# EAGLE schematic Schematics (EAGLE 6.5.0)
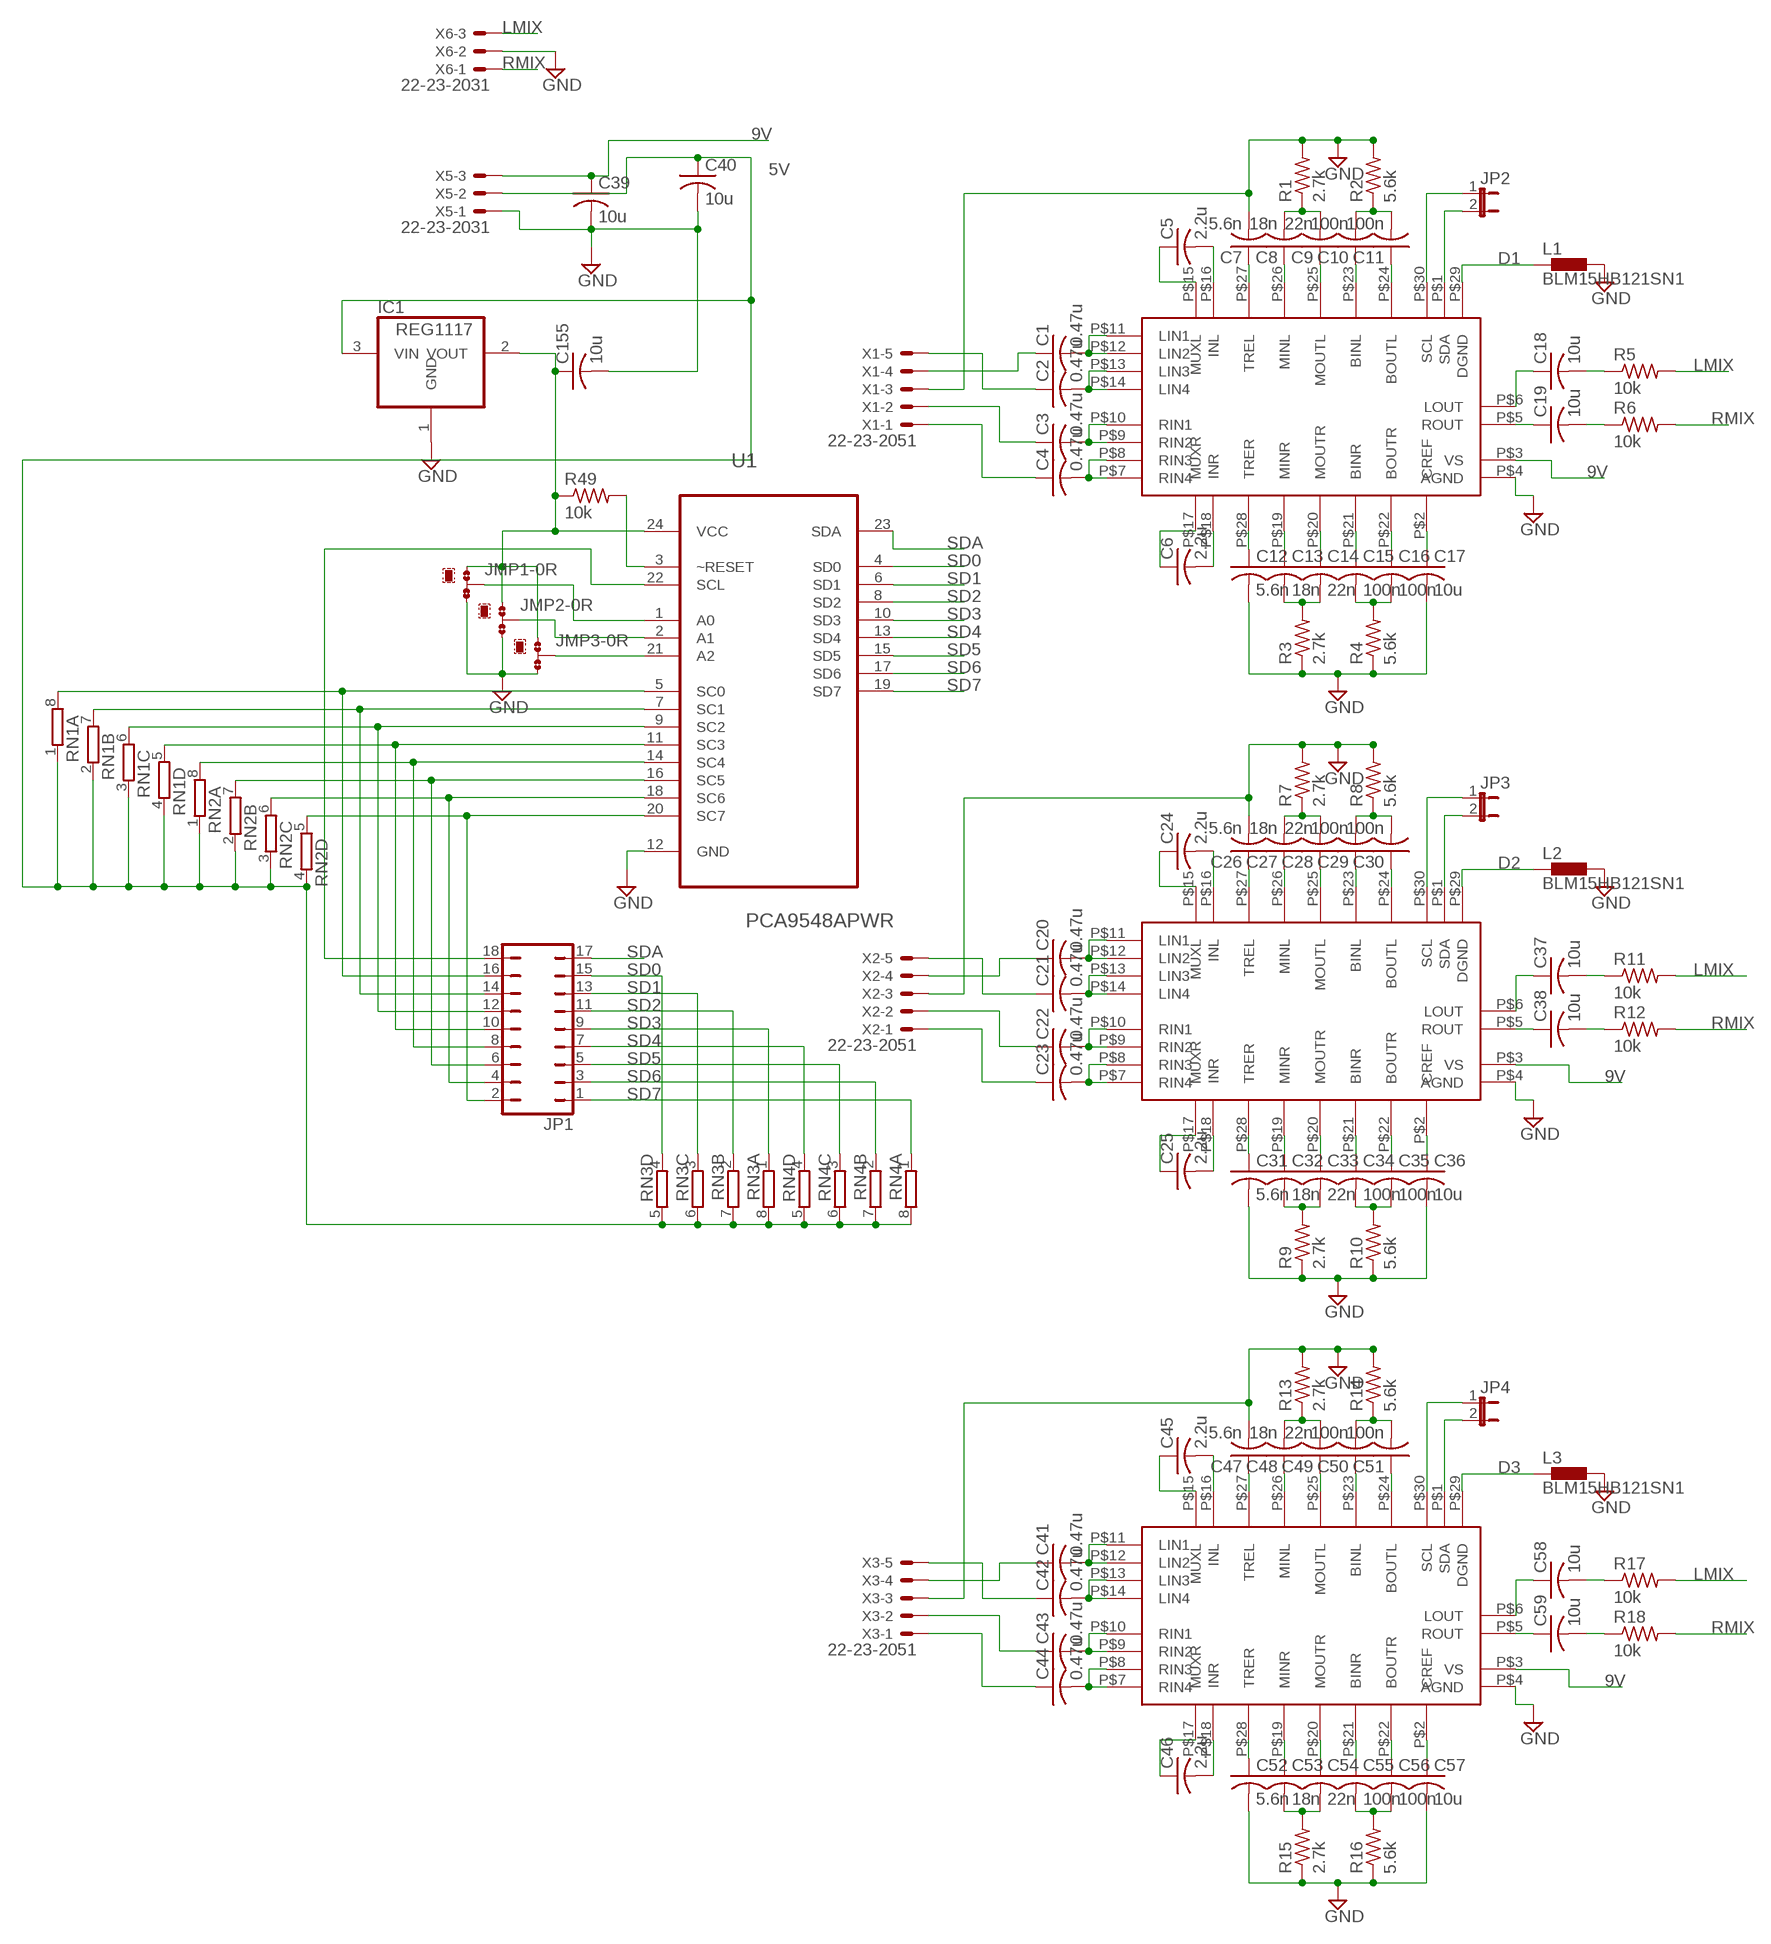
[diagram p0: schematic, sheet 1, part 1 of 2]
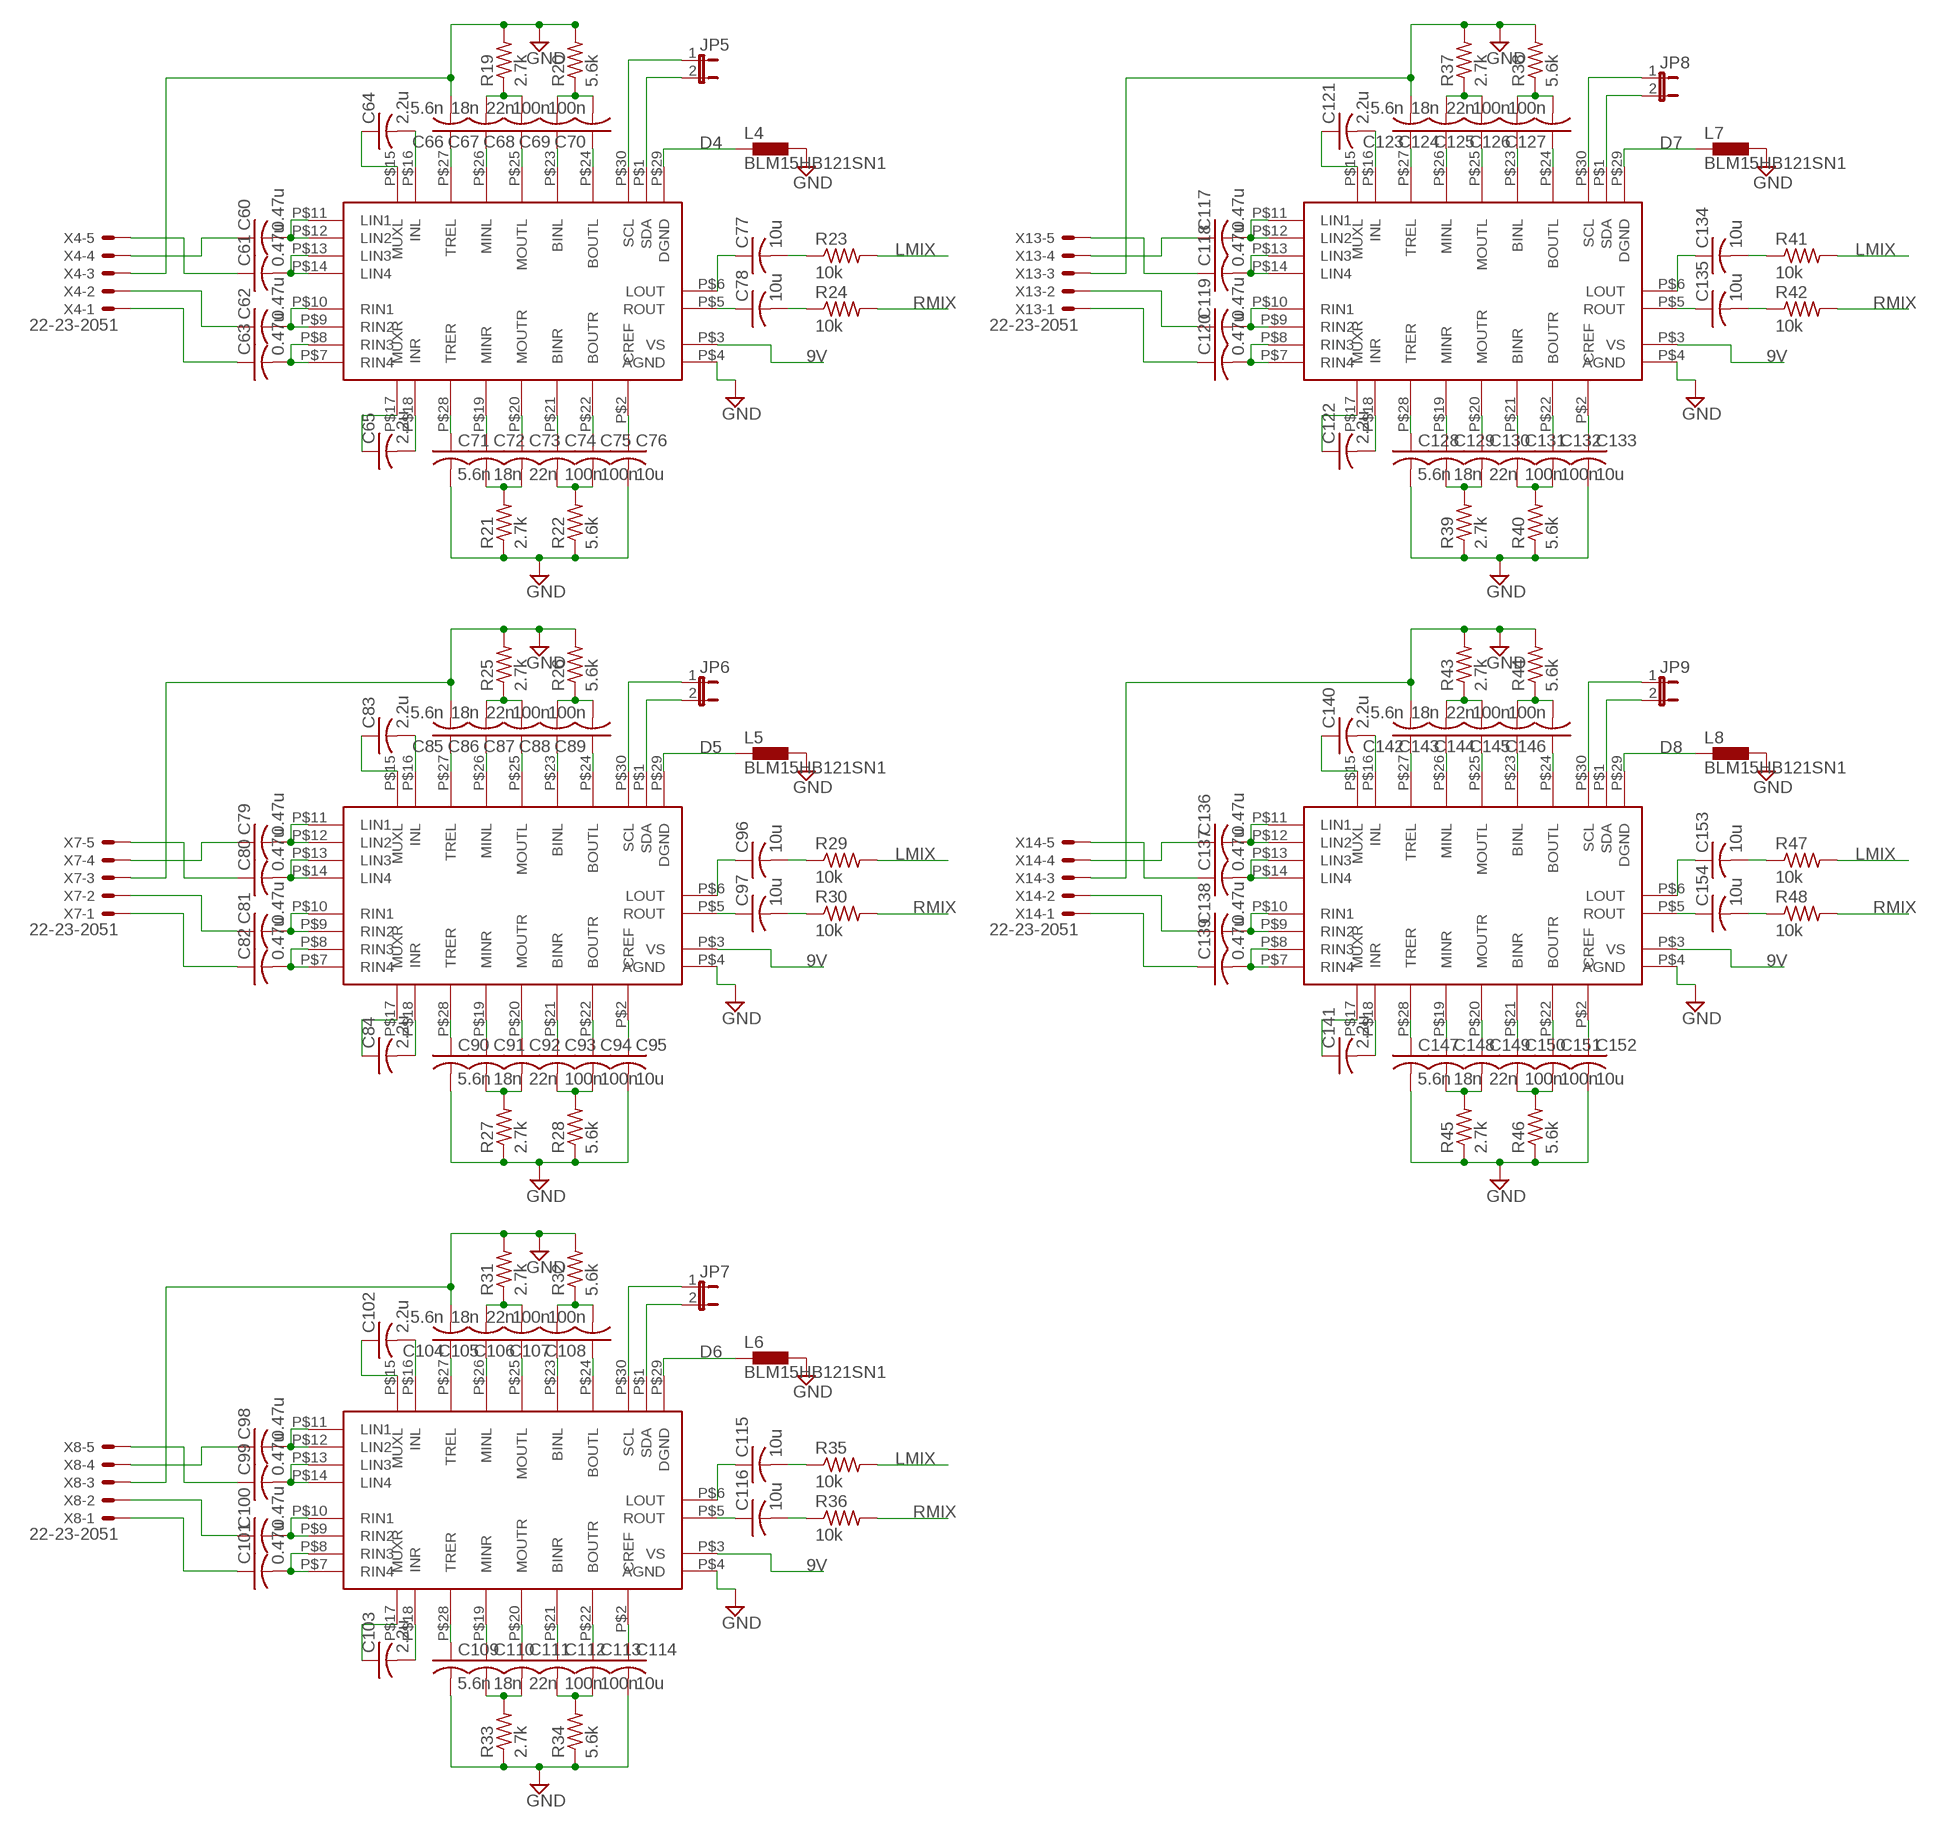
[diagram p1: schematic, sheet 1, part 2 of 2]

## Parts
C1  0.47u  C-USC1206  [C1206]
C2  0.47u  C-USC1206  [C1206]
C3  0.47u  C-USC1206  [C1206]
C4  0.47u  C-USC1206  [C1206]
C5  2.2u  C-USC1206  [C1206]
C6  2.2u  C-USC1206  [C1206]
C7  5.6n  C-USC1206  [C1206]
C8  18n  C-USC1206  [C1206]
C9  22n  C-USC1206  [C1206]
C10  100n  C-USC1206  [C1206]
C11  100n  C-USC1206  [C1206]
C12  5.6n  C-USC1206  [C1206]
C13  18n  C-USC1206  [C1206]
C14  22n  C-USC1206  [C1206]
C15  100n  C-USC1206  [C1206]
C16  100n  C-USC1206  [C1206]
C17  10u  C-USC1206  [C1206]
C18  10u  C-USC1206  [C1206]
C19  10u  C-USC1206  [C1206]
C20  0.47u  C-USC1206  [C1206]
C21  0.47u  C-USC1206  [C1206]
C22  0.47u  C-USC1206  [C1206]
C23  0.47u  C-USC1206  [C1206]
C24  2.2u  C-USC1206  [C1206]
C25  2.2u  C-USC1206  [C1206]
C26  5.6n  C-USC1206  [C1206]
C27  18n  C-USC1206  [C1206]
C28  22n  C-USC1206  [C1206]
C29  100n  C-USC1206  [C1206]
C30  100n  C-USC1206  [C1206]
C31  5.6n  C-USC1206  [C1206]
C32  18n  C-USC1206  [C1206]
C33  22n  C-USC1206  [C1206]
C34  100n  C-USC1206  [C1206]
C35  100n  C-USC1206  [C1206]
C36  10u  C-USC1206  [C1206]
C37  10u  C-USC1206  [C1206]
C38  10u  C-USC1206  [C1206]
C39  10u  C-USC1206  [C1206]
C40  10u  C-USC1206  [C1206]
C41  0.47u  C-USC1206  [C1206]
C42  0.47u  C-USC1206  [C1206]
C43  0.47u  C-USC1206  [C1206]
C44  0.47u  C-USC1206  [C1206]
C45  2.2u  C-USC1206  [C1206]
C46  2.2u  C-USC1206  [C1206]
C47  5.6n  C-USC1206  [C1206]
C48  18n  C-USC1206  [C1206]
C49  22n  C-USC1206  [C1206]
C50  100n  C-USC1206  [C1206]
C51  100n  C-USC1206  [C1206]
C52  5.6n  C-USC1206  [C1206]
C53  18n  C-USC1206  [C1206]
C54  22n  C-USC1206  [C1206]
C55  100n  C-USC1206  [C1206]
C56  100n  C-USC1206  [C1206]
C57  10u  C-USC1206  [C1206]
C58  10u  C-USC1206  [C1206]
C59  10u  C-USC1206  [C1206]
C60  0.47u  C-USC1206  [C1206]
C61  0.47u  C-USC1206  [C1206]
C62  0.47u  C-USC1206  [C1206]
C63  0.47u  C-USC1206  [C1206]
C64  2.2u  C-USC1206  [C1206]
C65  2.2u  C-USC1206  [C1206]
C66  5.6n  C-USC1206  [C1206]
C67  18n  C-USC1206  [C1206]
C68  22n  C-USC1206  [C1206]
C69  100n  C-USC1206  [C1206]
C70  100n  C-USC1206  [C1206]
C71  5.6n  C-USC1206  [C1206]
C72  18n  C-USC1206  [C1206]
C73  22n  C-USC1206  [C1206]
C74  100n  C-USC1206  [C1206]
C75  100n  C-USC1206  [C1206]
C76  10u  C-USC1206  [C1206]
C77  10u  C-USC1206  [C1206]
C78  10u  C-USC1206  [C1206]
C79  0.47u  C-USC1206  [C1206]
C80  0.47u  C-USC1206  [C1206]
C81  0.47u  C-USC1206  [C1206]
C82  0.47u  C-USC1206  [C1206]
C83  2.2u  C-USC1206  [C1206]
C84  2.2u  C-USC1206  [C1206]
C85  5.6n  C-USC1206  [C1206]
C86  18n  C-USC1206  [C1206]
C87  22n  C-USC1206  [C1206]
C88  100n  C-USC1206  [C1206]
C89  100n  C-USC1206  [C1206]
C90  5.6n  C-USC1206  [C1206]
C91  18n  C-USC1206  [C1206]
C92  22n  C-USC1206  [C1206]
C93  100n  C-USC1206  [C1206]
C94  100n  C-USC1206  [C1206]
C95  10u  C-USC1206  [C1206]
C96  10u  C-USC1206  [C1206]
C97  10u  C-USC1206  [C1206]
C98  0.47u  C-USC1206  [C1206]
C99  0.47u  C-USC1206  [C1206]
C100  0.47u  C-USC1206  [C1206]
C101  0.47u  C-USC1206  [C1206]
C102  2.2u  C-USC1206  [C1206]
C103  2.2u  C-USC1206  [C1206]
C104  5.6n  C-USC1206  [C1206]
C105  18n  C-USC1206  [C1206]
C106  22n  C-USC1206  [C1206]
C107  100n  C-USC1206  [C1206]
C108  100n  C-USC1206  [C1206]
C109  5.6n  C-USC1206  [C1206]
C110  18n  C-USC1206  [C1206]
C111  22n  C-USC1206  [C1206]
C112  100n  C-USC1206  [C1206]
C113  100n  C-USC1206  [C1206]
C114  10u  C-USC1206  [C1206]
C115  10u  C-USC1206  [C1206]
C116  10u  C-USC1206  [C1206]
C117  0.47u  C-USC1206  [C1206]
C118  0.47u  C-USC1206  [C1206]
C119  0.47u  C-USC1206  [C1206]
C120  0.47u  C-USC1206  [C1206]
C121  2.2u  C-USC1206  [C1206]
C122  2.2u  C-USC1206  [C1206]
C123  5.6n  C-USC1206  [C1206]
C124  18n  C-USC1206  [C1206]
C125  22n  C-USC1206  [C1206]
C126  100n  C-USC1206  [C1206]
C127  100n  C-USC1206  [C1206]
C128  5.6n  C-USC1206  [C1206]
C129  18n  C-USC1206  [C1206]
C130  22n  C-USC1206  [C1206]
C131  100n  C-USC1206  [C1206]
C132  100n  C-USC1206  [C1206]
C133  10u  C-USC1206  [C1206]
C134  10u  C-USC1206  [C1206]
C135  10u  C-USC1206  [C1206]
C136  0.47u  C-USC1206  [C1206]
C137  0.47u  C-USC1206  [C1206]
C138  0.47u  C-USC1206  [C1206]
C139  0.47u  C-USC1206  [C1206]
C140  2.2u  C-USC1206  [C1206]
C141  2.2u  C-USC1206  [C1206]
C142  5.6n  C-USC1206  [C1206]
C143  18n  C-USC1206  [C1206]
C144  22n  C-USC1206  [C1206]
C145  100n  C-USC1206  [C1206]
C146  100n  C-USC1206  [C1206]
C147  5.6n  C-USC1206  [C1206]
C148  18n  C-USC1206  [C1206]
C149  22n  C-USC1206  [C1206]
C150  100n  C-USC1206  [C1206]
C151  100n  C-USC1206  [C1206]
C152  10u  C-USC1206  [C1206]
C153  10u  C-USC1206  [C1206]
C154  10u  C-USC1206  [C1206]
C155  10u  C-USC1206  [C1206]
IC1  REG1117  [SOT223]
JMP1  0R-JUMPB  [B0R-JMP]
JMP2  0R-JUMPB  [B0R-JMP]
JMP3  0R-JUMPB  [B0R-JMP]
JP1  JP9Q  [JP9Q]
JP2  JP1E  [JP1]
JP3  JP1E  [JP1]
JP4  JP1E  [JP1]
JP5  JP1E  [JP1]
JP6  JP1E  [JP1]
JP7  JP1E  [JP1]
JP8  JP1E  [JP1]
JP9  JP1E  [JP1]
L1  BLM15HB121SN1  [0402]
L2  BLM15HB121SN1  [0402]
L3  BLM15HB121SN1  [0402]
L4  BLM15HB121SN1  [0402]
L5  BLM15HB121SN1  [0402]
L6  BLM15HB121SN1  [0402]
L7  BLM15HB121SN1  [0402]
L8  BLM15HB121SN1  [0402]
R1  2.7k  R-US_M1206  [M1206]
R2  5.6k  R-US_M1206  [M1206]
R3  2.7k  R-US_M1206  [M1206]
R4  5.6k  R-US_M1206  [M1206]
R5  10k  R-US_R1206  [R1206]
R6  10k  R-US_R1206  [R1206]
R7  2.7k  R-US_M1206  [M1206]
R8  5.6k  R-US_M1206  [M1206]
R9  2.7k  R-US_M1206  [M1206]
R10  5.6k  R-US_M1206  [M1206]
R11  10k  R-US_R1206  [R1206]
R12  10k  R-US_R1206  [R1206]
R13  2.7k  R-US_M1206  [M1206]
R14  5.6k  R-US_M1206  [M1206]
R15  2.7k  R-US_M1206  [M1206]
R16  5.6k  R-US_M1206  [M1206]
R17  10k  R-US_R1206  [R1206]
R18  10k  R-US_R1206  [R1206]
R19  2.7k  R-US_M1206  [M1206]
R20  5.6k  R-US_M1206  [M1206]
R21  2.7k  R-US_M1206  [M1206]
R22  5.6k  R-US_M1206  [M1206]
R23  10k  R-US_R1206  [R1206]
R24  10k  R-US_R1206  [R1206]
R25  2.7k  R-US_M1206  [M1206]
R26  5.6k  R-US_M1206  [M1206]
R27  2.7k  R-US_M1206  [M1206]
R28  5.6k  R-US_M1206  [M1206]
R29  10k  R-US_R1206  [R1206]
R30  10k  R-US_R1206  [R1206]
R31  2.7k  R-US_M1206  [M1206]
R32  5.6k  R-US_M1206  [M1206]
R33  2.7k  R-US_M1206  [M1206]
R34  5.6k  R-US_M1206  [M1206]
R35  10k  R-US_R1206  [R1206]
R36  10k  R-US_R1206  [R1206]
R37  2.7k  R-US_M1206  [M1206]
R38  5.6k  R-US_M1206  [M1206]
R39  2.7k  R-US_M1206  [M1206]
R40  5.6k  R-US_M1206  [M1206]
R41  10k  R-US_R1206  [R1206]
R42  10k  R-US_R1206  [R1206]
R43  2.7k  R-US_M1206  [M1206]
R44  5.6k  R-US_M1206  [M1206]
R45  2.7k  R-US_M1206  [M1206]
R46  5.6k  R-US_M1206  [M1206]
R47  10k  R-US_R1206  [R1206]
R48  10k  R-US_R1206  [R1206]
R49  10k  R-US_R1206  [R1206]
RN1  4R-NCAY16  [CAY16]
RN2  4R-NCAY16  [CAY16]
RN3  4R-NCAY16  [CAY16]
RN4  4R-NCAY16  [CAY16]
U1  PCA9548APWR  [SOP65P640X120-24N]
U$1  TDA7439  [SDIP30]
U$2  TDA7439  [SDIP30]
U$3  TDA7439  [SDIP30]
U$4  TDA7439  [SDIP30]
U$5  TDA7439  [SDIP30]
U$6  TDA7439  [SDIP30]
U$7  TDA7439  [SDIP30]
U$8  TDA7439  [SDIP30]
X1  22-23-2051  [22-23-2051]
X2  22-23-2051  [22-23-2051]
X3  22-23-2051  [22-23-2051]
X4  22-23-2051  [22-23-2051]
X5  22-23-2031  [22-23-2031]
X6  22-23-2031  [22-23-2031]
X7  22-23-2051  [22-23-2051]
X8  22-23-2051  [22-23-2051]
X13  22-23-2051  [22-23-2051]
X14  22-23-2051  [22-23-2051]

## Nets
5V: C40.1 IC1.3(VIN) RN1.1 RN1.2 RN1.3 RN1.4 RN2.1 RN2.2 RN2.3 RN2.4 RN3.5 RN3.6 RN3.7 RN3.8 RN4.5 RN4.6 RN4.7 RN4.8 X5.2
9V: C39.1 U$1.P$3(VS) U$2.P$3(VS) U$3.P$3(VS) U$4.P$3(VS) U$5.P$3(VS) U$6.P$3(VS) U$7.P$3(VS) U$8.P$3(VS) X5.3
D1: L1.1 U$1.P$29(DGND)
D2: L2.1 U$2.P$29(DGND)
D3: L3.1 U$3.P$29(DGND)
D4: L4.1 U$4.P$29(DGND)
D5: L5.1 U$5.P$29(DGND)
D6: L6.1 U$6.P$29(DGND)
D7: L7.1 U$7.P$29(DGND)
D8: L8.1 U$8.P$29(DGND)
GND: C7.2 C12.2 C17.2 C26.2 C31.2 C36.2 C39.2 C40.2 C47.2 C52.2 C57.2 C66.2 C71.2 C76.2 C85.2 C90.2 C95.2 C104.2 C109.2 C114.2 C123.2 C128.2 C133.2 C142.2 C147.2 C152.2 C155.2 IC1.1(GND) JMP1.3 JMP2.3 JMP3.3 L1.2 L2.2 L3.2 L4.2 L5.2 L6.2 L7.2 L8.2 R1.2 R2.2 R3.1 R4.1 R7.2 R8.2 R9.1 R10.1 R13.2 R14.2 R15.1 R16.1 R19.2 R20.2 R21.1 R22.1 R25.2 R26.2 R27.1 R28.1 R31.2 R32.2 R33.1 R34.1 R37.2 R38.2 R39.1 R40.1 R43.2 R44.2 R45.1 R46.1 U1.12(GND) U$1.P$4(AGND) U$2.P$4(AGND) U$3.P$4(AGND) U$4.P$4(AGND) U$5.P$4(AGND) U$6.P$4(AGND) U$7.P$4(AGND) U$8.P$4(AGND) X1.3 X2.3 X3.3 X4.3 X5.1 X6.2 X7.3 X8.3 X13.3 X14.3
LMIX: R5.2 R11.2 R17.2 R23.2 R29.2 R35.2 R41.2 R47.2 X6.3
N$1: C1.1 X1.4
N$2: C1.2 U$1.P$11(LIN1) U$1.P$12(LIN2)
N$3: C2.1 X1.5
N$4: C2.2 U$1.P$13(LIN3) U$1.P$14(LIN4)
N$5: C3.1 X1.2
N$6: C3.2 U$1.P$9(RIN2) U$1.P$10(RIN1)
N$7: C4.1 X1.1
N$8: C4.2 U$1.P$7(RIN4) U$1.P$8(RIN3)
N$9: C5.1 U$1.P$15(MUXL)
N$10: C5.2 U$1.P$16(INL)
N$11: C6.1 U$1.P$17(MUXR)
N$12: C6.2 U$1.P$18(INR)
N$13: C7.1 U$1.P$27(TREL)
N$14: C8.1 U$1.P$26(MINL)
N$15: C9.1 U$1.P$25(MOUTL)
N$16: C10.1 U$1.P$23(BINL)
N$17: C11.1 U$1.P$24(BOUTL)
N$18: C12.1 U$1.P$28(TRER)
N$19: C13.1 U$1.P$19(MINR)
N$20: C14.1 U$1.P$20(MOUTR)
N$21: C15.1 U$1.P$21(BINR)
N$22: C16.1 U$1.P$22(BOUTR)
N$23: C17.1 U$1.P$2(CREF)
N$24: C8.2 C9.2 R1.1
N$25: C10.2 C11.2 R2.1
N$26: C13.2 C14.2 R3.2
N$27: C15.2 C16.2 R4.2
N$28: R49.2 U1.3(~RESET)
N$29: C18.1 U$1.P$6(LOUT)
N$30: C19.1 U$1.P$5(ROUT)
N$31: C18.2 R5.1
N$32: C19.2 R6.1
N$33: C20.2 U$2.P$11(LIN1) U$2.P$12(LIN2)
N$34: C21.2 U$2.P$13(LIN3) U$2.P$14(LIN4)
N$35: C22.2 U$2.P$9(RIN2) U$2.P$10(RIN1)
N$36: C23.2 U$2.P$7(RIN4) U$2.P$8(RIN3)
N$37: C24.1 U$2.P$15(MUXL)
N$38: C24.2 U$2.P$16(INL)
N$39: C25.1 U$2.P$17(MUXR)
N$40: C25.2 U$2.P$18(INR)
N$41: C26.1 U$2.P$27(TREL)
N$42: C27.1 U$2.P$26(MINL)
N$43: C28.1 U$2.P$25(MOUTL)
N$44: C29.1 U$2.P$23(BINL)
N$45: C30.1 U$2.P$24(BOUTL)
N$46: C31.1 U$2.P$28(TRER)
N$47: C32.1 U$2.P$19(MINR)
N$48: C33.1 U$2.P$20(MOUTR)
N$49: C34.1 U$2.P$21(BINR)
N$50: C35.1 U$2.P$22(BOUTR)
N$51: C36.1 U$2.P$2(CREF)
N$52: C27.2 C28.2 R7.1
N$53: C29.2 C30.2 R8.1
N$54: C32.2 C33.2 R9.2
N$55: C34.2 C35.2 R10.2
N$56: C37.1 U$2.P$6(LOUT)
N$57: C38.1 U$2.P$5(ROUT)
N$58: C37.2 R11.1
N$59: C38.2 R12.1
N$60: C21.1 X2.5
N$61: C20.1 X2.4
N$62: C22.1 X2.2
N$63: C23.1 X2.1
N$64: C41.2 U$3.P$11(LIN1) U$3.P$12(LIN2)
N$65: C42.2 U$3.P$13(LIN3) U$3.P$14(LIN4)
N$66: C43.2 U$3.P$9(RIN2) U$3.P$10(RIN1)
N$67: C44.2 U$3.P$7(RIN4) U$3.P$8(RIN3)
N$68: C45.1 U$3.P$15(MUXL)
N$69: C45.2 U$3.P$16(INL)
N$70: C46.1 U$3.P$17(MUXR)
N$71: C46.2 U$3.P$18(INR)
N$72: C47.1 U$3.P$27(TREL)
N$73: C48.1 U$3.P$26(MINL)
N$74: C49.1 U$3.P$25(MOUTL)
N$75: C50.1 U$3.P$23(BINL)
N$76: C51.1 U$3.P$24(BOUTL)
N$77: C52.1 U$3.P$28(TRER)
N$78: C53.1 U$3.P$19(MINR)
N$79: C54.1 U$3.P$20(MOUTR)
N$80: C55.1 U$3.P$21(BINR)
N$81: C56.1 U$3.P$22(BOUTR)
N$82: C57.1 U$3.P$2(CREF)
N$83: C48.2 C49.2 R13.1
N$84: C50.2 C51.2 R14.1
N$85: C53.2 C54.2 R15.2
N$86: C55.2 C56.2 R16.2
N$87: C58.1 U$3.P$6(LOUT)
N$88: C59.1 U$3.P$5(ROUT)
N$89: C58.2 R17.1
N$90: C59.2 R18.1
N$91: C43.1 X3.2
N$92: C44.1 X3.1
N$93: C42.1 X3.5
N$94: C41.1 X3.4
N$95: C60.2 U$4.P$11(LIN1) U$4.P$12(LIN2)
N$96: C61.2 U$4.P$13(LIN3) U$4.P$14(LIN4)
N$97: C62.2 U$4.P$9(RIN2) U$4.P$10(RIN1)
N$98: C63.2 U$4.P$7(RIN4) U$4.P$8(RIN3)
N$99: C64.1 U$4.P$15(MUXL)
N$100: C64.2 U$4.P$16(INL)
N$101: C65.1 U$4.P$17(MUXR)
N$102: C65.2 U$4.P$18(INR)
N$103: C66.1 U$4.P$27(TREL)
N$104: C67.1 U$4.P$26(MINL)
N$105: C68.1 U$4.P$25(MOUTL)
N$106: C69.1 U$4.P$23(BINL)
N$107: C70.1 U$4.P$24(BOUTL)
N$108: C71.1 U$4.P$28(TRER)
N$109: C72.1 U$4.P$19(MINR)
N$110: C73.1 U$4.P$20(MOUTR)
N$111: C74.1 U$4.P$21(BINR)
N$112: C75.1 U$4.P$22(BOUTR)
N$113: C76.1 U$4.P$2(CREF)
N$114: C67.2 C68.2 R19.1
N$115: C69.2 C70.2 R20.1
N$116: C72.2 C73.2 R21.2
N$117: C74.2 C75.2 R22.2
N$118: C77.1 U$4.P$6(LOUT)
N$119: C78.1 U$4.P$5(ROUT)
N$120: C77.2 R23.1
N$121: C78.2 R24.1
N$122: C62.1 X4.2
N$123: C63.1 X4.1
N$124: C61.1 X4.5
N$125: C60.1 X4.4
N$126: C79.2 U$5.P$11(LIN1) U$5.P$12(LIN2)
N$127: C80.2 U$5.P$13(LIN3) U$5.P$14(LIN4)
N$128: C81.2 U$5.P$9(RIN2) U$5.P$10(RIN1)
N$129: C82.2 U$5.P$7(RIN4) U$5.P$8(RIN3)
N$130: C83.1 U$5.P$15(MUXL)
N$131: C83.2 U$5.P$16(INL)
N$132: C84.1 U$5.P$17(MUXR)
N$133: C84.2 U$5.P$18(INR)
N$134: C85.1 U$5.P$27(TREL)
N$135: C86.1 U$5.P$26(MINL)
N$136: C87.1 U$5.P$25(MOUTL)
N$137: C88.1 U$5.P$23(BINL)
N$138: C89.1 U$5.P$24(BOUTL)
N$139: C90.1 U$5.P$28(TRER)
N$140: C91.1 U$5.P$19(MINR)
N$141: C92.1 U$5.P$20(MOUTR)
N$142: C93.1 U$5.P$21(BINR)
N$143: C94.1 U$5.P$22(BOUTR)
N$144: C95.1 U$5.P$2(CREF)
N$145: C86.2 C87.2 R25.1
N$146: C88.2 C89.2 R26.1
N$147: C91.2 C92.2 R27.2
N$148: C93.2 C94.2 R28.2
N$149: C96.1 U$5.P$6(LOUT)
N$150: C97.1 U$5.P$5(ROUT)
N$151: C96.2 R29.1
N$152: C97.2 R30.1
N$153: C81.1 X7.2
N$154: C82.1 X7.1
N$155: C80.1 X7.5
N$156: C79.1 X7.4
N$157: C98.2 U$6.P$11(LIN1) U$6.P$12(LIN2)
N$158: C99.2 U$6.P$13(LIN3) U$6.P$14(LIN4)
N$159: C100.2 U$6.P$9(RIN2) U$6.P$10(RIN1)
N$160: C101.2 U$6.P$7(RIN4) U$6.P$8(RIN3)
N$161: C102.1 U$6.P$15(MUXL)
N$162: C102.2 U$6.P$16(INL)
N$163: C103.1 U$6.P$17(MUXR)
N$164: C103.2 U$6.P$18(INR)
N$165: C104.1 U$6.P$27(TREL)
N$166: C105.1 U$6.P$26(MINL)
N$167: C106.1 U$6.P$25(MOUTL)
N$168: C107.1 U$6.P$23(BINL)
N$169: C108.1 U$6.P$24(BOUTL)
N$170: C109.1 U$6.P$28(TRER)
N$171: C110.1 U$6.P$19(MINR)
N$172: C111.1 U$6.P$20(MOUTR)
N$173: C112.1 U$6.P$21(BINR)
N$174: C113.1 U$6.P$22(BOUTR)
N$175: C114.1 U$6.P$2(CREF)
N$176: C105.2 C106.2 R31.1
N$177: C107.2 C108.2 R32.1
N$178: C110.2 C111.2 R33.2
N$179: C112.2 C113.2 R34.2
N$180: C115.1 U$6.P$6(LOUT)
N$181: C116.1 U$6.P$5(ROUT)
N$182: C115.2 R35.1
N$183: C116.2 R36.1
N$184: C100.1 X8.2
N$185: C101.1 X8.1
N$186: C99.1 X8.5
N$187: C98.1 X8.4
N$188: C117.2 U$7.P$11(LIN1) U$7.P$12(LIN2)
N$189: C118.2 U$7.P$13(LIN3) U$7.P$14(LIN4)
N$190: C119.2 U$7.P$9(RIN2) U$7.P$10(RIN1)
N$191: C120.2 U$7.P$7(RIN4) U$7.P$8(RIN3)
N$192: C121.1 U$7.P$15(MUXL)
N$193: C121.2 U$7.P$16(INL)
N$194: C122.1 U$7.P$17(MUXR)
N$195: C122.2 U$7.P$18(INR)
N$196: C123.1 U$7.P$27(TREL)
N$197: C124.1 U$7.P$26(MINL)
N$198: C125.1 U$7.P$25(MOUTL)
N$199: C126.1 U$7.P$23(BINL)
N$200: C127.1 U$7.P$24(BOUTL)
N$201: C128.1 U$7.P$28(TRER)
N$202: C129.1 U$7.P$19(MINR)
N$203: C130.1 U$7.P$20(MOUTR)
N$204: C131.1 U$7.P$21(BINR)
N$205: C132.1 U$7.P$22(BOUTR)
N$206: C133.1 U$7.P$2(CREF)
N$207: C124.2 C125.2 R37.1
N$208: C126.2 C127.2 R38.1
N$209: C129.2 C130.2 R39.2
N$210: C131.2 C132.2 R40.2
N$211: C134.1 U$7.P$6(LOUT)
N$212: C135.1 U$7.P$5(ROUT)
N$213: C134.2 R41.1
N$214: C135.2 R42.1
N$215: C119.1 X13.2
N$216: C120.1 X13.1
N$217: C118.1 X13.5
N$218: C117.1 X13.4
N$219: C136.2 U$8.P$11(LIN1) U$8.P$12(LIN2)
N$220: C137.2 U$8.P$13(LIN3) U$8.P$14(LIN4)
N$221: C138.2 U$8.P$9(RIN2) U$8.P$10(RIN1)
N$222: C139.2 U$8.P$7(RIN4) U$8.P$8(RIN3)
N$223: C140.1 U$8.P$15(MUXL)
N$224: C140.2 U$8.P$16(INL)
N$225: C141.1 U$8.P$17(MUXR)
N$226: C141.2 U$8.P$18(INR)
N$227: C142.1 U$8.P$27(TREL)
N$228: C143.1 U$8.P$26(MINL)
N$229: C144.1 U$8.P$25(MOUTL)
N$230: C145.1 U$8.P$23(BINL)
N$231: C146.1 U$8.P$24(BOUTL)
N$232: C147.1 U$8.P$28(TRER)
N$233: C148.1 U$8.P$19(MINR)
N$234: C149.1 U$8.P$20(MOUTR)
N$235: C150.1 U$8.P$21(BINR)
N$236: C151.1 U$8.P$22(BOUTR)
N$237: C152.1 U$8.P$2(CREF)
N$238: C143.2 C144.2 R43.1
N$239: C145.2 C146.2 R44.1
N$240: C148.2 C149.2 R45.2
N$241: C150.2 C151.2 R46.2
N$242: C153.1 U$8.P$6(LOUT)
N$243: C154.1 U$8.P$5(ROUT)
N$244: C153.2 R47.1
N$245: C154.2 R48.1
N$246: C138.1 X14.2
N$247: C139.1 X14.1
N$248: C137.1 X14.5
N$249: C136.1 X14.4
N$250: JP1.2 RN2.5 U1.20(SC7)
N$251: JP1.4 RN2.6 U1.18(SC6)
N$252: JP1.6 RN2.7 U1.16(SC5)
N$253: JP1.8 RN2.8 U1.14(SC4)
N$254: JP1.10 RN1.5 U1.11(SC3)
N$255: JP1.12 RN1.6 U1.9(SC2)
N$256: JP1.14 RN1.7 U1.7(SC1)
N$257: JP1.18 U1.22(SCL)
N$258: JP2.1 U$1.P$30(SCL)
N$259: JP1.16 RN1.8 U1.5(SC0)
N$260: JP2.2 U$1.P$1(SDA)
N$261: JP3.1 U$2.P$30(SCL)
N$262: JP3.2 U$2.P$1(SDA)
N$263: JP4.1 U$3.P$30(SCL)
N$264: JP4.2 U$3.P$1(SDA)
N$265: JP5.1 U$4.P$30(SCL)
N$266: JP5.2 U$4.P$1(SDA)
N$267: JP6.1 U$5.P$30(SCL)
N$268: JP6.2 U$5.P$1(SDA)
N$269: JP7.1 U$6.P$30(SCL)
N$270: JP7.2 U$6.P$1(SDA)
N$271: JP8.1 U$7.P$30(SCL)
N$272: JP8.2 U$7.P$1(SDA)
N$273: JP9.1 U$8.P$30(SCL)
N$274: JP9.2 U$8.P$1(SDA)
N$275: JMP1.2 U1.1(A0)
N$276: JMP2.2 U1.2(A1)
N$277: JMP3.2 U1.21(A2)
N$278: C155.1 IC1.2(VOUT) JMP1.1 JMP2.1 JMP3.1 R49.1 U1.24(VCC)
RMIX: R6.2 R12.2 R18.2 R24.2 R30.2 R36.2 R42.2 R48.2 X6.1
SD0: JP1.15 RN3.4 U1.4(SD0)
SD1: JP1.13 RN3.3 U1.6(SD1)
SD2: JP1.11 RN3.2 U1.8(SD2)
SD3: JP1.9 RN3.1 U1.10(SD3)
SD4: JP1.7 RN4.4 U1.13(SD4)
SD5: JP1.5 RN4.3 U1.15(SD5)
SD6: JP1.3 RN4.2 U1.17(SD6)
SD7: JP1.1 RN4.1 U1.19(SD7)
SDA: JP1.17 U1.23(SDA)

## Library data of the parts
C1-C155 = adafruit:C-US: CAPACITOR, American symbol
IC1 = burr-brown:REG1117: 800mA and 1A Low Dropout (LDO) Positive Regulator 1.8V, 2.5V, 2.85V, 3.3V, 5V, and Adj; MPN: REG1117; OC_FARNELL: 1097566; OC_NEWARK: 14P6981
JMP1-JMP3 = jump-0r-smd:0R-JUMP: SMD 0R 0805 Jumper
JP1 = jumper:JP9Q: JUMPER
JP2-JP9 = jumper:JP1E: JUMPER
L1-L8 = inductors:BLM15H: EMIFIL (R) Chip Ferrite Bead for GHz Noise
R1-R49 = adafruit:R-US_: RESISTOR, American symbol
RN1-RN4 = resistor-dil:4R-N: Array Chip Resistor Source: RS Component / Phycomp; OC_FARNELL: unknown; OC_NEWARK: unknown
U1 = PCA9548A:PCA9548APWR: 8-CHANNEL I2C SWITCH WITH RESET; MPN: PCA9548APWR False; OC_FARNELL: 1607855; OC_NEWARK: 22M1602; PACKAGE: TSSOP-24; SUPPLIER: Texas Instruments
U$1-U$8 = adafruit:TDA7439
X1-X4 X7 X8 X13 X14 = con-molex:22-23-2051: .100" (2.54mm) Center Header - 5 Pin; MF: MOLEX; MPN: 22-23-2051; OC_FARNELL: 1462952; OC_NEWARK: 38C9178
X5 X6 = con-molex:22-23-2031: .100" (2.54mm) Center Header - 3 Pin; MF: MOLEX; MPN: 22-23-2031; OC_FARNELL: 1462950; OC_NEWARK: 30C0862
